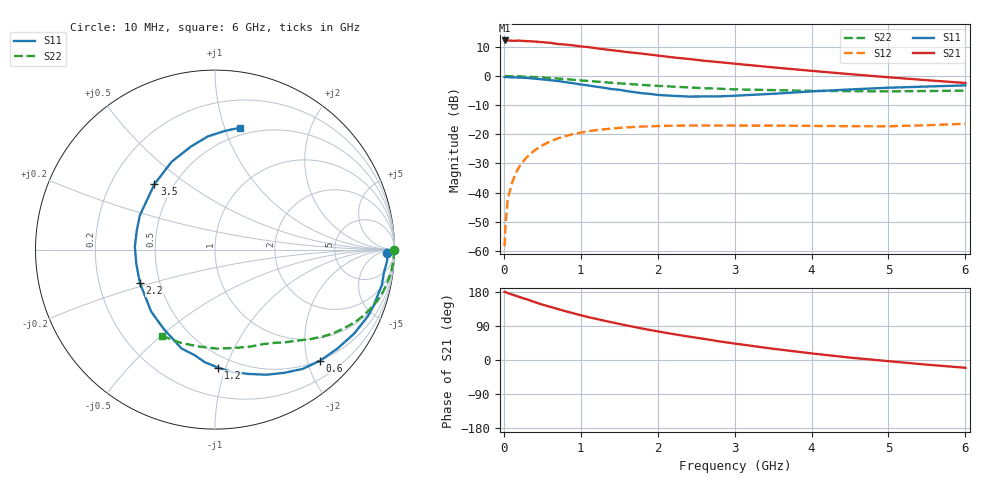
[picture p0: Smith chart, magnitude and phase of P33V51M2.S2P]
! SIEMENS Small Signal Semiconductors
! BFP181
! Si NPN RF Bipolar Junction Transistor in SOT143
! VCE = 3.5 V  IC = 1.2 mA
! Common Emitter S-Parameters:  March  1996
# GHz  S  MA  R  50
!  f  S11  S21  S12  S22
! GHz  MAG  ANG  MAG  ANG  MAG  ANG  MAG  ANG
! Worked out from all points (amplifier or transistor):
!   36 points, 10 MHz to 6 GHz, reference 50 ohm
!   highest |S21| = 12.2 dB at 10 MHz (marker M1)
!   |S21| within 3 dB of that: start of sweep to 1.298 GHz
!   unconditionally stable (mu >= 1): 2.939 GHz to end of sweep
!   at 250 MHz: K = 0.10, MSG = 20.7 dB, |S12| = -29.4 dB
!   at 1.4 GHz: K = 0.53, MSG = 13.5 dB, |S12| = -18.0 dB
!   at 6 GHz: K = 1.24, MAG = 4.0 dB, |S12| = -16.4 dB
!   S11 on the Smith chart (normalised r, x): 10 MHz: 40, -16; 600 MHz: 0.49, -2.23; 1.2 GHz: 0.41, -0.94; 2.2 GHz: 0.39, -0.18; 3.5 GHz: 0.39, +0.38; 6 GHz: 0.43, +1.13
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0.01  0.9582 -1.0  4.094 179.5  0.0012 88.6  0.9981 -0.2
0.02  0.9607 -1.7  4.073 179.2  0.0027 93.7  0.9979 -0.8
0.05  0.9609 -3.8  4.083 176.7  0.0075 91.9  0.9964 -1.9
0.1  0.9495 -7.9  4.055 173.3  0.0138 83.0  0.9969 -3.7
0.15  0.9507 -12.0  4.039 169.8  0.0209 82.7  0.9911 -5.5
0.2  0.9414 -15.9  4.069 166.3  0.0278 79.9  0.9893 -7.2
0.4  0.9053 -31.2  3.924 152.9  0.0532 70.1  0.9646 -14.3
0.6  0.8518 -46.6  3.734 140.4  0.0754 60.2  0.9271 -20.7
0.9  0.7541 -67.6  3.374 123.4  0.1012 48.3  0.8655 -28.7
1.1  0.6901 -81.8  3.149 113.0  0.1135 41.6  0.824 -33.3
1.2  0.6578 -88.4  3.009 108.6  0.1181 38.3  0.805 -35.5
1.5  0.5822 -108.6  2.699 95.2  0.1288 30.6  0.7496 -40.9
1.7  0.529 -122.0  2.509 87.0  0.134 26.4  0.7204 -44.1
1.9  0.4954 -136.0  2.342 79.2  0.1369 22.4  0.6918 -47.0
2.2  0.4583 -155.8  2.093 68.5  0.1406 17.8  0.6591 -51.2
2.4  0.4457 -169.6  1.973 61.9  0.1416 14.9  0.6395 -54.1
2.8  0.4486 166.3  1.735 49.2  0.1418 10.7  0.607 -59.6
3.5  0.4968 132.8  1.412 29.7  0.1413 5.6  0.5749 -70.1
4  0.5457 116.3  1.232 17.4  0.1395 3.5  0.5582 -79.2
4.5  0.5898 103.1  1.08 6.3  0.1379 2.4  0.5513 -89.3
5.5  0.6619 85.6  0.85 -12.3  0.1434 4.3  0.5537 -110.4
6  0.6929 78.5  0.762 -20.5  0.1519 4.3  0.5638 -121.4
